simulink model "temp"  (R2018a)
settings: Solver=FixedStepDiscrete  StartTime=0.0  StopTime=inf  RelTol=1e-3  EnableMultiTasking=on
libraries: arduinolib x2, dsparch4 x1

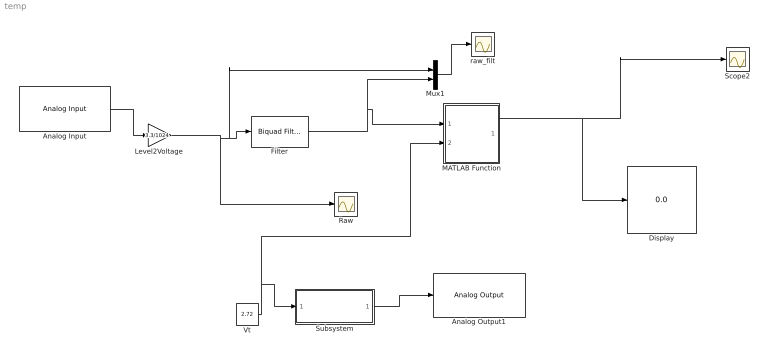
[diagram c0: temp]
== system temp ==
  Analog Input : arduinolib/Analog Input  pinNumber=5  ReadResultsOnly=off  ConversionTriggerSource=Software  ExternalTriggerType=uint32(0)  OutputDataType=uint16  EnableConversionCompleteNotify=off  EnableOuputStatus=off  SampleTime=0.01  blockPlatform=arduino
  Analog Output1 : arduinolib/Analog Output  DACpin=DAC1  blockPlatform=arduino
  Display : Display
  Filter : dsparch4/Biquad Filter  Tag=BlockMethodSubSystem  IIRFiltStruct=Direct form II  CoeffSource=Specify via dialog  BiQuadCoeffs=[1 2 1 1 -1.17564273339370851 0.590215815099901175;1 2 1 1 -0.911519710238840486 0.232953700834604677]  a0Flag=Warning  IC=0  ICnum=0  ICden=0  InputProcessing=Columns as channels (frame based)  denAccumFracLength=30  denProdOutputFracLength=30  secondMemoryFracLength=15  roundingMode=Floor  overflowMode=off  ScaleValues=[0.10364327042654814;0.0803584976489410407;1]  optimizeScaleValues=on  ScaleValueMode=Specify via input port (g)  scaleValueFracLength=14  FilterSource=Specify via dialog  FilterObject=BQF
  "Level2Voltage " : Gain  Gain=3.3/1024  OutDataTypeStr=double
  MATLAB Function : MATLAB Function  TreatAsAtomicUnit=on
  Mux1 : Mux  Inputs=2
  Raw : Scope
  Scope2 : Scope
  Subsystem : Subsystem
  Vt : Constant  Value=2.72  OutDataTypeStr=double
  raw_filt : Scope
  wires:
  MATLAB Function/1(out) -> Display/1, Scope2/1
  "Level2Voltage "/1 -> Mux1/1, Filter/1, Raw/1
  Filter/1 -> MATLAB Function/1(v), Mux1/2
  Mux1/1 -> raw_filt/1
  Analog Input/1 -> "Level2Voltage "/1
  Vt/1 -> Subsystem/1(In1), MATLAB Function/2(o)
  Subsystem/1(Out1) -> Analog Output1/1

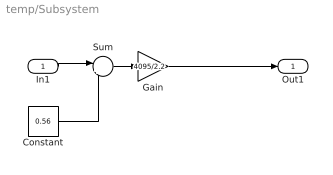
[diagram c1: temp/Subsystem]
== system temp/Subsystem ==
  In1 : Inport
  Constant : Constant  Value=0.56
  Gain : Gain  Gain=4095/2.2  OutDataTypeStr=uint16
  Sum : Sum  Inputs=|+-
  Out1 : Outport
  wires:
  In1/1 -> Sum/1
  Constant/1 -> Sum/2
  Sum/1 -> Gain/1
  Gain/1 -> Out1/1

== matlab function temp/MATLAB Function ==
function out  = fcn(v,o)

TCR=-3950/ (273+25)^2;

out=(v-o)*4/( 3.3 * TCR )+25;
